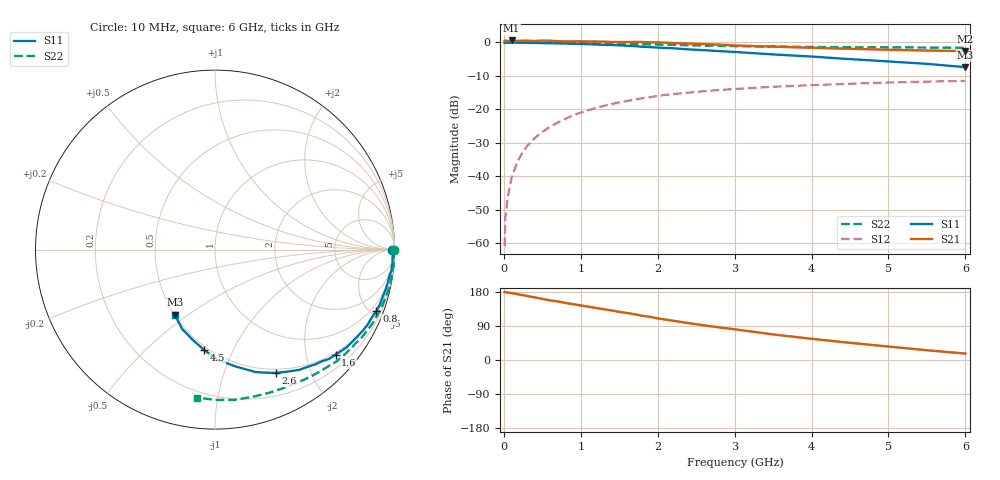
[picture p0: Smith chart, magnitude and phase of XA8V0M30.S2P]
! SIEMENS Discrete & RF Semiconductors
! BFY180
! Si NPN RF Bipolar Junction Transistor in MICRO-X
! VCE = 8 V  IC = 0.3 mA
! Common Emitter S-Parameters:  May  1997
# GHz  S  MA  R  50
!  f  S11  S21  S12  S22
! GHz  MAG  ANG  MAG  ANG  MAG  ANG  MAG  ANG
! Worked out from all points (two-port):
!   36 points, 10 MHz to 6 GHz, reference 50 ohm
!   highest |S21| = 0.58 dB at 100 MHz (marker M1); lowest = -2.6 dB at 6 GHz (marker M2)
!   |S21| within 3 dB of the highest: start of sweep to 5.457 GHz
!   lowest |S11| = -7.4 dB at 6 GHz (marker M3), VSWR 2.49, Z = 25.1 - j22.3 ohm
!   |S11| at or under -10 dB: nowhere
!   |S22| runs from -1.6 to 0.0 dB; largest |S21 - S12| = 1.1
!   S11 on the Smith chart (normalised r, x): 10 MHz: open; 800 MHz: 0.59, -5.39; 1.6 GHz: 0.46, -2.60; 2.6 GHz: 0.46, -1.51; 4.5 GHz: 0.48, -0.78; 6 GHz: 0.50, -0.45
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0.01  0.9888 -0.2  1.056 179.7  0.0009 91.8  0.9986 -0.2
0.02  0.9847 -0.4  1.062 179.0  0.0024 88.0  0.9999 -0.5
0.05  0.9921 -1.2  1.049 178.2  0.0048 81.7  0.9999 -1.1
0.1  0.9903 -2.6  1.069 176.5  0.0094 89.4  0.9969 -2.1
0.15  0.9922 -4.2  1.054 174.9  0.0137 86.9  0.9999 -3.1
0.2  0.9891 -5.3  1.054 172.8  0.0185 86.0  0.9993 -4.1
0.3  0.9841 -8.0  1.06 169.0  0.028 83.7  0.9972 -6.2
0.4  0.9804 -10.6  1.05 165.3  0.0371 81.1  0.9966 -8.2
0.5  0.9759 -13.4  1.064 161.4  0.0459 79.2  0.995 -10.3
0.6  0.9708 -15.6  1.059 157.2  0.0549 76.9  0.992 -12.3
0.8  0.9618 -20.8  1.034 150.6  0.0721 72.5  0.9857 -16.3
1.1  0.9399 -28.6  1.031 140.6  0.0969 65.8  0.9745 -22.3
1.6  0.8912 -41.1  1.013 124.0  0.1329 55.4  0.9488 -32.0
1.8  0.8604 -46.3  1.014 116.6  0.1465 51.8  0.9381 -35.5
2  0.8361 -51.0  1.001 109.7  0.1586 47.8  0.929 -39.1
2.2  0.8175 -55.1  0.977 103.6  0.1692 44.1  0.9202 -42.6
2.6  0.7653 -63.8  0.944 91.5  0.1865 37.7  0.8972 -48.9
3.5  0.6611 -80.0  0.865 67.5  0.2173 25.1  0.8649 -61.9
4  0.6143 -88.6  0.83 55.9  0.2298 19.0  0.8535 -68.8
4.5  0.5626 -96.1  0.802 45.3  0.2409 13.5  0.8469 -75.7
5.5  0.478 -112.6  0.755 25.7  0.2593 2.7  0.8376 -89.8
6  0.4263 -121.6  0.742 17.0  0.2655 -2.9  0.8303 -96.9
